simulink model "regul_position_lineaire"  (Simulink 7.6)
settings: Solver=ode15s  StartTime=0.0  StopTime=10.0  RelTol=1e-3
StopFcn:
  | close all
  | load consigne_cde_sortie.mat
  | plot(ccs(1,:),ccs(2,:),ccs(1,:),ccs(3,:),ccs(1,:),ccs(4,:))
  | title('Signaux de consigne, sortie et de commande')
  | xlabel('temps')
  | axis([0 10 -0.6 1.2])
  | %axis([0 10 -1.5 1.5])
  | grid
  | figure
  | plot(ccs(1,:),ccs(5,:))
  | title('Signal d''érreur')
  | grid
undefined symbols (not defined in the file or in its folder): sigbuilder_block
libraries: fl_lib x12, nesl_utility x5

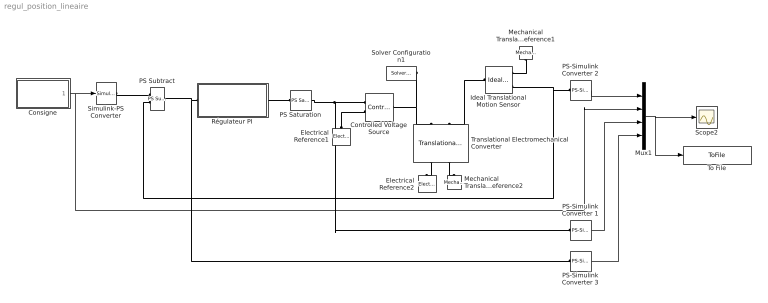
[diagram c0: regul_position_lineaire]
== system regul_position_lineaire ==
  Consigne : Subsystem  Tag=STV Subsys  LoadFcn=sigbuilder_block('load');  StartFcn=sigbuilder_block('start');  StopFcn=sigbuilder_block('stop');  ClipboardFcn=sigbuilder_block('clipboard');
  Controlled Voltage Source : fl_lib/Electrical/Electrical Sources/Controlled Voltage Source  DialogController=NetworkEngine.DynNeDlgSource  SystemSampleTime=-1  i_Log=off  v_Log=off  LocalVarNames=|i|v  LocalVarDescs=|i|v  LocalVarLogging=[0 0]
  Electrical Reference1 : fl_lib/Electrical/Electrical Elements/Electrical Reference  DialogController=NetworkEngine.DynNeDlgSource  SystemSampleTime=-1  i_Log=off  LocalVarNames=|i  LocalVarDescs=|i  LocalVarLogging=[]
  Electrical Reference2 : fl_lib/Electrical/Electrical Elements/Electrical Reference  DialogController=NetworkEngine.DynNeDlgSource  SystemSampleTime=-1  i_Log=off  LocalVarNames=|i  LocalVarDescs=|i  LocalVarLogging=[]
  Ideal Translational Motion Sensor : fl_lib/Mechanical/Mechanical Sensors/Ideal Translational Motion Sensor  DialogController=NetworkEngine.DynNeDlgSource  SystemSampleTime=-1  offset=0 m  v_Log=off  f_Log=off  x_Log=off  LocalVarNames=|v|f|x  LocalVarDescs=|v|f|x  LocalVarLogging=[0 0 0]
  Mechanical Translational Reference1 : fl_lib/Mechanical/Translational Elements/Mechanical Translational Reference  DialogController=NetworkEngine.DynNeDlgSource  SystemSampleTime=-1  f_Log=off  LocalVarNames=|f  LocalVarDescs=|f  LocalVarLogging=0
  Mechanical Translational Reference2 : fl_lib/Mechanical/Translational Elements/Mechanical Translational Reference  DialogController=NetworkEngine.DynNeDlgSource  SystemSampleTime=-1  f_Log=off  LocalVarNames=|f  LocalVarDescs=|f  LocalVarLogging=0
  Mux1 : Mux
  PS Saturation : fl_lib/Physical Signals/Nonlinear Operators/PS Saturation  DialogController=NetworkEngine.DynNeDlgSource  SystemSampleTime=-1  upper_limit=0.5  lower_limit=-0.5  LocalVarLogging=[]
  PS Subtract : fl_lib/Physical Signals/Functions/PS Subtract  DialogController=NetworkEngine.DynNeDlgSource  SystemSampleTime=-1  LocalVarLogging=[]
  PS-Simulink Converter 1 : nesl_utility/PS-Simulink Converter  DialogController=NetworkEngine.DynNeUtilDlgSource  SystemSampleTime=-1  PhysicalDomain=network_engine_domain  LeftPortType=input  RightPortType=output  SubClassName=ps_output  Unit=1  AffineConversion=off
  PS-Simulink Converter 2 : nesl_utility/PS-Simulink Converter  DialogController=NetworkEngine.DynNeUtilDlgSource  SystemSampleTime=-1  PhysicalDomain=network_engine_domain  LeftPortType=input  RightPortType=output  SubClassName=ps_output  Unit=m  AffineConversion=off
  PS-Simulink Converter 3 : nesl_utility/PS-Simulink Converter  DialogController=NetworkEngine.DynNeUtilDlgSource  SystemSampleTime=-1  PhysicalDomain=network_engine_domain  LeftPortType=input  RightPortType=output  SubClassName=ps_output  Unit=m  AffineConversion=off
  Régulateur PI : Subsystem  mask(Régulateur PI en composants physiques){K=1}
      mask prompts: K "Gain"
  Scope2 : Scope
  Simulink-PS Converter : nesl_utility/Simulink-PS Converter  DialogController=NetworkEngine.DynNeUtilDlgSource  SystemSampleTime=-1  PhysicalDomain=network_engine_domain  LeftPortType=input  RightPortType=output  SubClassName=ps_input  Unit=1  AffineConversion=off  InputFilterTimeConstant=.001  UdotUserProvided=0
  Solver Configuration1 : nesl_utility/Solver Configuration  DialogController=NetworkEngine.DynNeUtilDlgSource  SystemSampleTime=-1  PhysicalDomain=network_engine_domain  LeftPortType=input  RightPortType=generic  SubClassName=solver  Accelerate=off  Profile=off  ResidualTolerance=1e-9  MaxNonlinIter=12  MaxModeIter=2  DoFixedCost=off  UseLocalSampling=off  DoDC=off  LinearAlgebra=Sparse  LocalSolverSampleTime=.001  LocalSolverChoice=NE_BACKWARD_EULER_ADVANCER  UseLocalSolver=off
  To File : ToFile  Filename=consigne_cde_sortie  MatrixName=ccs
  Translational Electromechanical Converter : fl_lib/Electrical/Electrical Elements/Translational Electromechanical Converter  DialogController=NetworkEngine.DynNeDlgSource  SystemSampleTime=-1  K=0.1 s*V/m  i_Log=off  v_Log=off  f_Log=off  u_Log=off  LocalVarNames=|i|v|f|u  LocalVarDescs=|i|v|f|u  LocalVarLogging=[0 0 0 0]
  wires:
  Consigne/1(Signal 1) -> Simulink-PS Converter/1, Mux1/2
  Mux1/1 -> Scope2/1, To File/1
  PS-Simulink Converter 1/1 -> Mux1/3
  PS-Simulink Converter 2/1 -> Mux1/1
  PS-Simulink Converter 3/1 -> Mux1/4
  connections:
  Solver Configuration1/RConn1 -- Translational Electromechanical Converter/LConn1 -- Controlled Voltage Source/LConn1
  Ideal Translational Motion Sensor/LConn1 -- Translational Electromechanical Converter/LConn2
  Mechanical Translational Reference1/LConn1 -- Ideal Translational Motion Sensor/RConn1
  Simulink-PS Converter/RConn1 -- PS Subtract/LConn1
  PS Subtract/LConn2 -- Ideal Translational Motion Sensor/RConn3 -- PS-Simulink Converter 2/LConn1
  Translational Electromechanical Converter/RConn1 -- Electrical Reference2/LConn1
  Translational Electromechanical Converter/RConn2 -- Mechanical Translational Reference2/LConn1
  Electrical Reference1/LConn1 -- Controlled Voltage Source/RConn2
  PS-Simulink Converter 3/LConn1 -- PS Subtract/RConn1 -- Régulateur PI/LConn1
  Controlled Voltage Source/RConn1 -- PS-Simulink Converter 1/LConn1 -- PS Saturation/RConn1
  Régulateur PI/RConn1 -- PS Saturation/LConn1

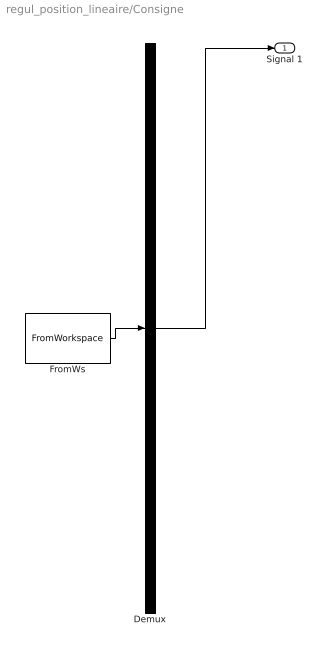
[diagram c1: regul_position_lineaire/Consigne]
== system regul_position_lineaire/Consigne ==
  Demux : Demux  Tag=STV Demux  Outputs=1
  FromWs : FromWorkspace  Tag=STV FromWs  VariableName=tuvar  SampleTime=0  SigBuilderData=DataTag0  VnvData=DataTag1
  Signal 1 : Outport  Tag=STV Outport
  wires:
  Demux/1 -> Signal 1/1
  FromWs/1 -> Demux/1

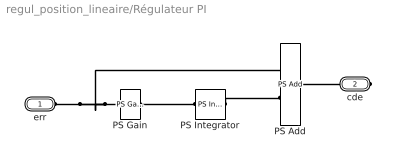
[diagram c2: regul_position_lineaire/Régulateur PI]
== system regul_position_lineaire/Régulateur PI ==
  PS Add : fl_lib/Physical Signals/Functions/PS Add  DialogController=NetworkEngine.DynNeDlgSource  SystemSampleTime=-1  LocalVarLogging=[]
  PS Gain : fl_lib/Physical Signals/Functions/PS Gain  DialogController=NetworkEngine.DynNeDlgSource  SystemSampleTime=-1  gain=K  LocalVarLogging=[]
  PS Integrator : fl_lib/Physical Signals/Linear Operators/PS Integrator  DialogController=NetworkEngine.DynNeDlgSource  SystemSampleTime=-1  x0=0  x_Log=off  LocalVarNames=|x  LocalVarDescs=|x  LocalVarLogging=0
  err : PMIOPort  Port=1  Side=Left
  cde : PMIOPort  Port=2  Side=Right
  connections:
  cde/RConn1 -- PS Add/RConn1
  PS Gain/RConn1 -- PS Integrator/LConn1
  PS Integrator/RConn1 -- PS Add/LConn2
  PS Gain/LConn1 -- err/RConn1 -- PS Add/LConn1
